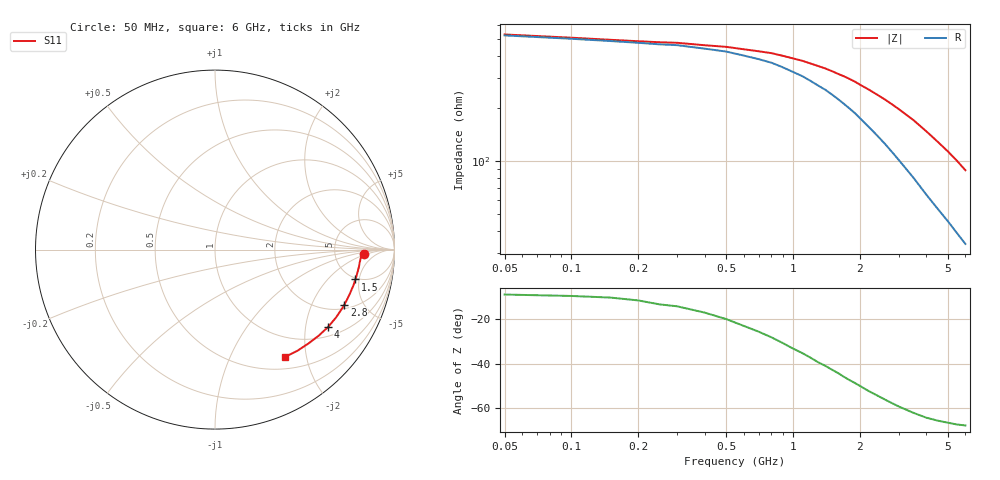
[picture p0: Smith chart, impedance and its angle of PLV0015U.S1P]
! Infineon Technologies  Discrete & RF Semiconductors
! BAR 64-04W /-05W /-06W
! Si PIN Diode in SOT323
! IF = 0.015 mA
! S-Parameters:  October  2008
# GHz  S  MA  R  50
!  f  S11
! GHz  MAG  ANG
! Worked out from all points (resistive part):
!   34 points, 50 MHz to 6 GHz, reference 50 ohm
!   read as one part to ground: R = 523 ohm at 50 MHz
!   S11 on the Smith chart (normalised r, x): 50 MHz: 10, -2; 1.5 GHz: 4.80, -4.43; 2.8 GHz: 2.25, -3.57; 4 GHz: 1.29, -2.66; 6 GHz: 0.67, -1.64
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0.05  0.8293 -1.7
0.1  0.8228 -1.9
0.15  0.8187 -2.1
0.2  0.8163 -2.4
0.25  0.8152 -2.8
0.3  0.8146 -3.0
0.4  0.8116 -3.7
0.5  0.811 -4.4
0.6  0.8092 -5.2
0.8  0.808 -6.6
1  0.8054 -8.2
1.1  0.8043 -8.9
1.3  0.8022 -10.5
1.4  0.8009 -11.2
1.5  0.7996 -12.0
1.6  0.798 -12.8
1.8  0.7968 -14.4
2.2  0.7912 -17.8
2.4  0.7882 -19.5
2.6  0.7859 -21.2
2.8  0.7831 -23.0
3  0.7805 -24.8
3.5  0.773 -29.4
4  0.7632 -34.5
4.5  0.7508 -39.7
5  0.7385 -45.0
5.5  0.7272 -50.7
6  0.7141 -56.8
